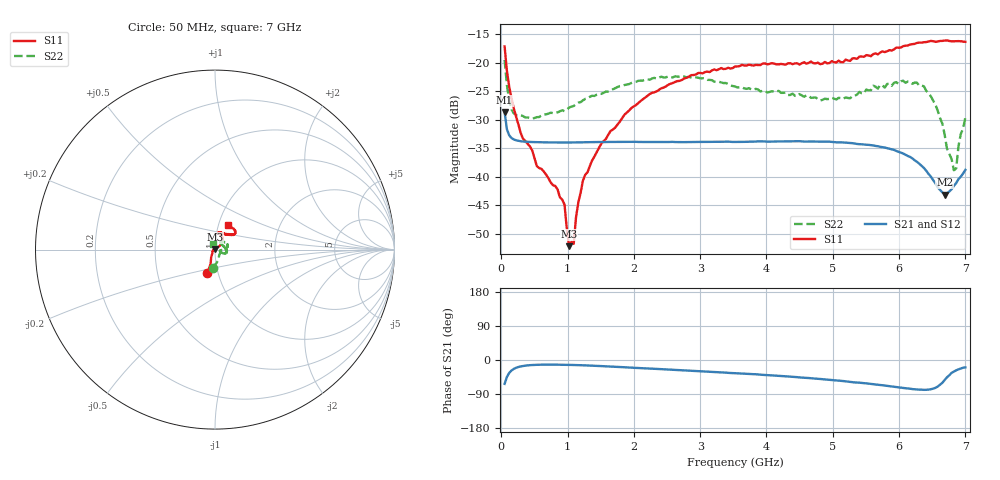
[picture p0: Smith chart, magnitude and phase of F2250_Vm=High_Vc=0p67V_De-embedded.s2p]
! Integrated Device Technology
! Corporate Headquarters
! 6024 Silver Creek Valley Road
! San Jose, CA 95138  USA
! Phone:  1-408-284-8200
! Toll Free:  1-800-223-1366
! Webpage:  http://www.idt.com/
! Timing and RF Division
! 515 Groton Road, Suite 102
! Westford, MA 01886-6024
! Device:  F2250
! Description: Voltage Variable RF Attenuator
! Frequency:  50.0 -  6000.00 MHz
! Package:  3x3 mm Thin QFN Plastic Package: 16 pin
! Ports:  2 RF, 3 DC
!  Pin  1  = GND
!  Pin  2  = NC
!  Pin  3  = RF1  = Port 1
!  Pin  4  = NC
!  Pin  5  = GND
!  Pin  6  = GND
!  Pin  7  = GND
!  Pin  8  = GND
!  Pin  9  = NC
!  Pin 10  = RF2  = Port 2
!  Pin 11  = NC
!  Pin 12  = GND
!  Pin 13  = GND
!  Pin 14  = VCNTRL
!  Pin 15  = VDD
!  Pin 16  = VMODE
! Vcntrl:  0.670 Volts
! Vmode:  +3.300 Volts
! Vdd:  +3.30  Volts
! Current:  1.282 mA
! Data:  The device was measured on a the F2250 evaluation board which has
!  individual transmission lines to the RF pins.  Data was collected
!  using a calibrated network analyzer.  The evaluation board was
!  de-embedded using a TRL calibration technique.
!  The reference plane is the edge of the package pin.
! Misc:  SN 10
!  Action Tracker AT0258
! Date Measured:  2014-11-26
! Date:  2015-10-15  MJV
! Note:
!  Integrated Device Technology supplies this data as a sample of measured
!  data at the package pin for this product.  Your particular data for this
!  product may vary.
!  Data was taken at 25 degrees C.
!  Integrated Device Technology reserves the right to change this data at anytime.
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# GHz S dB R 50
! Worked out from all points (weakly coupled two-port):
!   201 points, 50 MHz to 7 GHz, reference 50 ohm
!   highest |S21| = -28.68 dB at 50 MHz (marker M1); lowest = -43.1 dB at 6.687 GHz (marker M2)
!   lowest |S11| = -52.1 dB at 1.023 GHz (marker M3), VSWR 1.00, Z = 49.8 + j0.167 ohm
!   |S11| at or under -10 dB: start of sweep to end of sweep
!   |S22| runs from -38.8 to -19.5 dB; largest |S21 - S12| = 6.3e-05
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0.05  -17.16 -108.2  -28.68 -63.0  -28.68 -63.0  -19.53 -96.5
0.1195  -24.20 -111.5  -32.72 -34.0  -32.72 -34.0  -26.64 -62.3
0.22375  -29.47 -121.7  -33.60 -20.5  -33.59 -20.5  -29.20 -38.3
0.5365  -38.13 -153.5  -33.93 -12.7  -33.93 -12.7  -29.54 -9.2
0.9535  -44.86 171.5  -33.99 -12.7  -33.98 -12.7  -28.51 -2.5
1.023  -52.14 137.2  -33.98 -12.9  -33.97 -12.9  -27.85 -1.3
1.0925  -51.73 81.3  -33.98 -13.2  -33.97 -13.2  -27.59 -0.1
1.12725  -47.05 55.4  -33.97 -13.3  -33.96 -13.4  -27.25 -0.7
1.2315  -40.66 38.2  -33.93 -13.9  -33.93 -13.9  -26.59 -1.3
1.6485  -31.97 40.2  -33.89 -17.2  -33.89 -17.2  -24.93 5.8
2.37825  -24.75 46.2  -33.89 -23.8  -33.89 -23.9  -22.65 15.8
3.525  -20.68 71.5  -33.88 -34.7  -33.88 -34.7  -24.17 42.8
4.7065  -20.09 71.9  -33.81 -48.7  -33.81 -48.7  -26.12 49.1
5.2625  -19.69 53.1  -34.06 -57.7  -34.05 -57.8  -26.23 23.0
5.85325  -17.81 40.4  -35.09 -68.9  -35.08 -69.0  -23.67 -4.2
6.3745  -16.41 40.8  -38.44 -78.7  -38.45 -78.8  -24.14 -20.7
6.54825  -16.36 44.6  -41.14 -73.4  -41.17 -73.4  -27.34 -25.1
6.68725  -16.13 47.7  -43.13 -53.0  -43.13 -52.9  -32.60 -9.2
6.82625  -16.25 52.5  -41.58 -30.6  -41.55 -30.6  -38.84 58.7
6.861  -16.24 54.4  -41.09 -27.2  -41.07 -27.2  -38.54 69.8
6.89575  -16.23 56.4  -40.39 -24.7  -40.35 -24.6  -34.63 84.3
7  -16.35 62.3  -38.78 -19.5  -38.76 -19.6  -29.55 113.2
